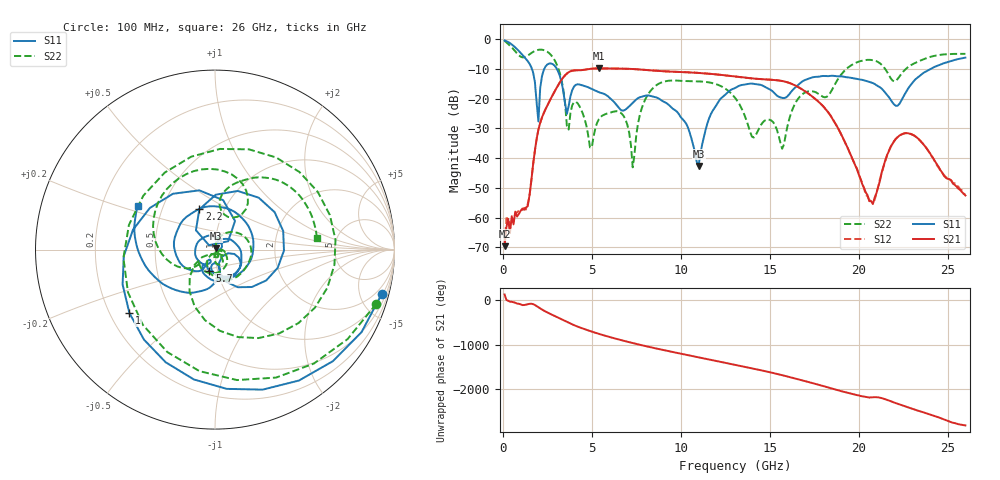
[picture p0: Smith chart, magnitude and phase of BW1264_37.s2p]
!Keysight Technologies,N5245B,MY57181159,A.13.60.06
!Date: Friday, December 18, 2020 23:53:59
!Correction: S11(Full 2 Port(1,2))
!S21(Full 2 Port(1,2))
!S12(Full 2 Port(1,2))
!S22(Full 2 Port(1,2))
!S2P File: Measurements: S11, S21, S12, S22:
# Hz S  dB  R 50
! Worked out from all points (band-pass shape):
!   260 points, 100 MHz to 26 GHz, reference 50 ohm
!   highest |S21| = -9.76 dB at 5.4 GHz (marker M1); lowest = -69.7 dB at 100 MHz (marker M2)
!   |S21| within 3 dB of the highest: 3.403 GHz to 13.4 GHz (10 GHz wide, 119 % of centre)
!   lowest |S11| = -42.6 dB at 11 GHz (marker M3), VSWR 1.01, Z = 50.4 + j0.634 ohm
!   |S11| at or under -10 dB: 1.638 GHz to 2.324 GHz (686.1 MHz wide, 34.6 % of centre); 3.04 GHz to 24.02 GHz (20.98 GHz wide, 155 % of centre)
!   |S22| runs from -43.1 to -0.5 dB; largest |S21 - S12| = 0.00057
!   S11 on the Smith chart (normalised r, x): 100 MHz: 1.14, -7.43; 1 GHz: 0.28, -0.31; 2.2 GHz: 0.76, +0.36; 5.7 GHz: 0.92, -0.22; 26 GHz: 0.36, +0.23
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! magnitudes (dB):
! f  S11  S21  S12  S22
! 100 MHz  -0.3  -69.7  -69.1  -0.5
! 1 GHz  -4.5  -57.8  -57.7  -5.8
! 2 GHz  -27.6  -30.4  -30.4  -3.5
! 2.2 GHz  -12.4  -26.3  -26.3  -3.5
! 3.1 GHz  -10.7  -15.5  -15.5  -9.5
! 3.7 GHz  -22.4  -11.1  -11.1  -30.4
! 4.5 GHz  -15.5  -10.3  -10.3  -25.1
! 4.9 GHz  -16.4  -9.9  -9.9  -36.4
! 5.4 GHz  -17.8  -9.8  -9.8  -26.9
! 5.7 GHz  -18.4  -9.8  -9.8  -25.4
! 6.8 GHz  -24.0  -9.9  -9.9  -25.9
! 7.3 GHz  -21.4  -10.0  -10.0  -43.1
! 7.8 GHz  -19.3  -10.2  -10.2  -23.3
! 8.8 GHz  -20.1  -10.6  -10.6  -14.8
! 11 GHz  -42.6  -11.3  -11.3  -14.1
! 13.1 GHz  -16.2  -12.5  -12.5  -20.0
! 15.7 GHz  -19.7  -14.0  -14.0  -36.8
! 17.4 GHz  -12.8  -19.3  -19.3  -17.5
! 20.8 GHz  -14.7  -55.5  -54.3  -7.0
! 21.7 GHz  -19.4  -37.6  -37.5  -12.0
! 23.1 GHz  -14.1  -32.3  -32.3  -8.1
! 26 GHz  -6.1  -52.6  -52.1  -4.9
